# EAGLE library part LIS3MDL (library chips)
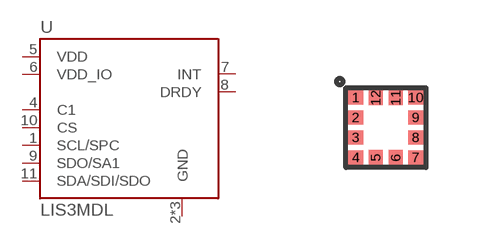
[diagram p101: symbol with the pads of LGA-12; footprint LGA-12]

Designator prefix U

## LIS3MDL (DIGIKEY: 497-13892-1-ND; MANUFACTURER: STM; MPN: LIS3MDLTR)  [LGA-12]
1  SCL/SPC
2  GND
3  GND
4  C1
5  VDD
6  VDD_IO
7  INT
8  DRDY
9  SDO/SA1
10  CS
11  SDA/SDI/SDO
12  GND

## Footprint LGA-12 (pad centres in mm)
smd 0.375 x 0.35: 1 -0.75,0.75; 2 -0.75,0.25; 3 -0.75,-0.25; 4 -0.75,-0.75; 7 0.75,-0.75; 8 0.75,-0.25; 9 0.75,0.25; 10 0.75,0.75
smd 0.35 x 0.375: 5 -0.25,-0.75; 6 0.25,-0.75; 11 0.25,0.75; 12 -0.25,0.75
